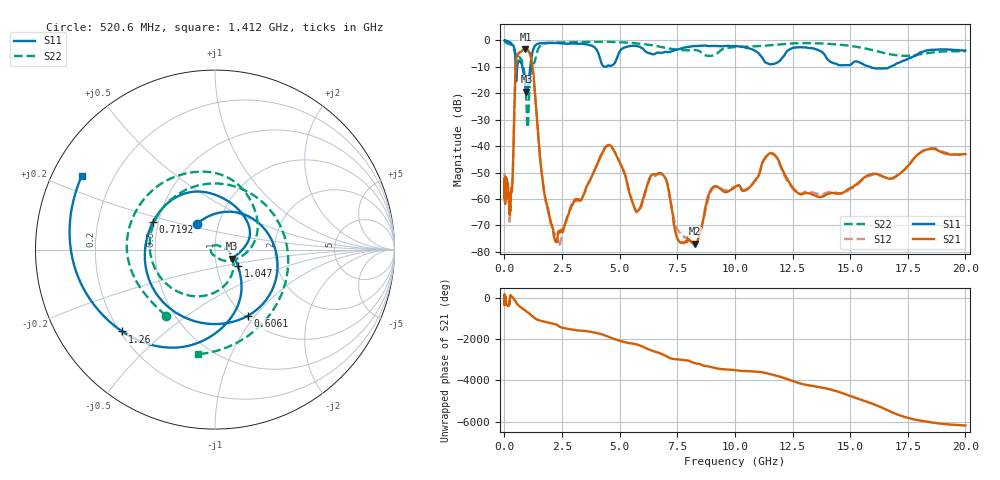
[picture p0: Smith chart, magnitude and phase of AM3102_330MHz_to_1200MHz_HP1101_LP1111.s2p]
! Date/Time: Tue, Sep 11, 2018 5:22 PM
! Network Analyzer: Agilent Technologies E8362B Rev: A.07.50.63
! Sweep from 0.010 to 20.000 GHz, 1601 Points, Sweep Type: LOG
! Power Supply: 4.949 V, 0.001 A
# Hz S DB R 50
!freq MagS11 AngS11 MagS21 AngS21 MagS12 AngS12 MagS22 AngS22
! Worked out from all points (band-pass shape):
!   1601 points, 10 MHz to 20 GHz, reference 50 ohm
!   highest |S21| = -3.24 dB at 916.3 MHz (marker M1); lowest = -77.0 dB at 8.266 GHz (marker M2)
!   |S21| within 3 dB of the highest: 527.3 MHz to 1.147 GHz (619.8 MHz wide, 74 % of centre)
!   lowest |S11| = -19.4 dB at 956.4 MHz (marker M3), VSWR 1.24, Z = 60.1 - j6.12 ohm
!   |S11| at or under -10 dB: 486.2 MHz to 557.9 MHz (71.73 MHz wide, 13.7 % of centre); 782.7 MHz to 1.12 GHz (337.2 MHz wide, 35.4 % of centre); 15.86 GHz to 16.74 GHz (877.8 MHz wide, 5.39 % of centre)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
!   |S22| runs from -33.0 to -0.2 dB; largest |S21 - S12| = 0.009
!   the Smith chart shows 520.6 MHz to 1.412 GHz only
!   S11 on the Smith chart (normalised r, x): 520.6 MHz: 0.78, +0.23; 606.1 MHz: 1.03, -0.92; 719.2 MHz: 0.47, +0.17; 1.047 GHz: 1.27, -0.24; 1.26 GHz: 0.21, -0.36; 1.412 GHz: 0.09, +0.26
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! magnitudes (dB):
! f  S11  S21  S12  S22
! 10 MHz  0.0  -58.2  -50.1  -0.2
! 35.55 MHz  -0.1  -59.9  -59.2  -0.5
! 126.4 MHz  -0.2  -54.3  -54.3  -1.1
! 235.5 MHz  -0.7  -65.4  -67.5  -1.4
! 351 MHz  -1.6  -53.2  -53.8  -2.3
! 447.2 MHz  -3.6  -21.5  -21.5  -4.1
! 520.6 MHz  -15.2  -6.6  -6.7  -6.8
! 606.1 MHz  -7.7  -5.0  -5.1  -6.1
! 719.2 MHz  -8.4  -4.2  -4.3  -7.0
! 916.3 MHz  -18.0  -3.2  -3.3  -17.4
! 956.4 MHz  -19.4  -3.3  -3.4  -23.6
! 1.047 GHz  -16.1  -4.0  -4.0  -27.7
! 1.26 GHz  -3.2  -13.2  -13.3  -8.7
! 1.412 GHz  -1.4  -29.8  -30.1  -4.6
! 1.59 GHz  -1.1  -48.0  -47.9  -1.8
! 2.336 GHz  -1.0  -72.8  -76.4  -0.8
! 4.479 GHz  -9.6  -39.8  -39.7  -0.5
! 5.652 GHz  -2.0  -63.6  -63.7  -1.0
! 6.771 GHz  -4.7  -50.2  -50.6  -2.4
! 8.266 GHz  -2.1  -77.0  -77.9  -3.6
! 11.53 GHz  -9.0  -42.7  -42.9  -1.8
! 20 GHz  -3.8  -43.0  -43.5  -4.1
